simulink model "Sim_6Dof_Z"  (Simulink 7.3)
settings: Solver=ode4  StartTime=0.0  StopTime=80  FixedStep=0.0005  MaxStep=0.0005  RelTol=1e-3
InitFcn:
  | run
StopFcn:
  | Pl
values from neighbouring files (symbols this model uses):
  calfa = cos(alfa0*d2r)    [run.m]
  d2r = pi/180    (= 0.0174532925199)    [run.m]
  salfa = sin(alfa0*d2r)    [run.m]
  Thet0 = 40    [run.m]
  V0 = 18640    [run.m]
undefined symbols (not defined in the file or in its folder): Acz, Avz, Bcz, Bvz, Ccz, Cvz, Dcz, DiscIntNeverNeededParam, Dvz
libraries: simulink x4

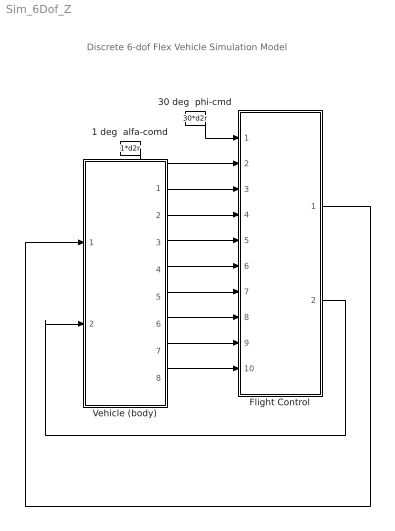
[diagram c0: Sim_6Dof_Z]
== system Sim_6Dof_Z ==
  note: Discrete 6-dof Flex Vehicle Simulation Model
  1 deg  alfa-comd : Constant  Value=1*d2r  OutDataType=sfix(16)  OutScaling=2^0
  30 deg  phi-cmd : Constant  Value=30*d2r  OutDataType=sfix(16)  OutScaling=2^0
  Flight Control : Subsystem
  Vehicle (body) : Subsystem
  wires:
  Vehicle (body)/1(phi) -> Flight Control/3(phi)
  Vehicle (body)/2(p) -> Flight Control/4(pb)
  Vehicle (body)/3(r) -> Flight Control/5(rb)
  Vehicle (body)/4(bet) -> Flight Control/6(beta)
  Vehicle (body)/5(theta) -> Flight Control/7(thet)
  Vehicle (body)/6(q) -> Flight Control/8(q)
  Vehicle (body)/7(alfa) -> Flight Control/9(alfa)
  Vehicle (body)/8(Nz) -> Flight Control/10(Nz)
  30 deg  phi-cmd/1 -> Flight Control/1(phi-cmd)
  1 deg  alfa-comd/1 -> Flight Control/2(alfa-cmd)
  Flight Control/2(Aer_pqr) -> Vehicle (body)/2(Aer_pqr)
  Flight Control/1(Jet_pqr) -> Vehicle (body)/1(Jet_pqr_Nz)

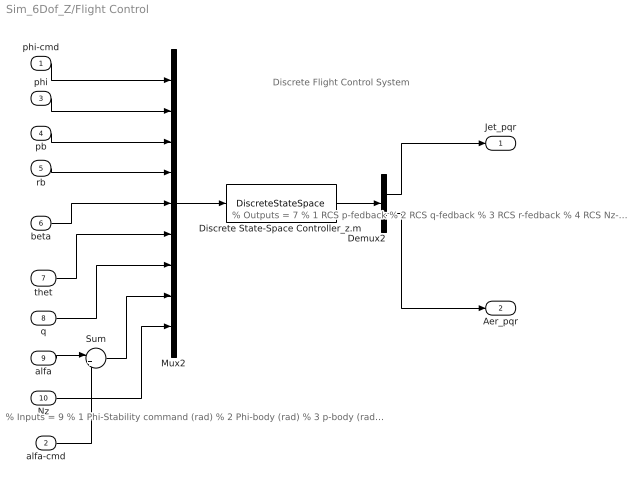
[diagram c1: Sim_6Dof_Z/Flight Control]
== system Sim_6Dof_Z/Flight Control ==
  note: Discrete Flight Control System
  note: % Outputs = 7 % 1 RCS p-fedback % 2 RCS q-fedback % 3 RCS r-fedback % 4 RCS Nz-fedback % 5 Aero-Surface p-feedback % 6 Aero-Surface q-feedback % 7 Aero-Surface r-feedback
  note: % Inputs = 9 % 1 Phi-Stability command (rad) % 2 Phi-body (rad) % 3 p-body (rad/sec) % 4 r-body (rad/sec) % 5 beta (rad) % 6 Theta (rad) % 7 q-body (rad/sec) % 8 alpha (rad) % 9 Nz (ft/sec^2)
  phi-cmd : Inport  OutDataType=sfix(16)  OutScaling=2^0
  alfa-cmd : Inport  Port=2  OutDataType=sfix(16)  OutScaling=2^0
  phi : Inport  Port=3  OutDataType=sfix(16)  OutScaling=2^0
  pb : Inport  Port=4  OutDataType=sfix(16)  OutScaling=2^0
  rb : Inport  Port=5  OutDataType=sfix(16)  OutScaling=2^0
  beta : Inport  Port=6  OutDataType=sfix(16)  OutScaling=2^0
  thet : Inport  Port=7  OutDataType=sfix(16)  OutScaling=2^0
  q : Inport  Port=8  OutDataType=sfix(16)  OutScaling=2^0
  alfa : Inport  Port=9  OutDataType=sfix(16)  OutScaling=2^0
  Nz : Inport  Port=10  OutDataType=sfix(16)  OutScaling=2^0
  Demux2 : Demux  Outputs=[4,3]
  Discrete State-Space Controller_z.m : DiscreteStateSpace  A=Acz  B=Bcz  C=Ccz  D=Dcz  SampleTime=0.04
  Mux2 : Mux  Inputs=9
  Sum : Sum  Inputs=|+-  OutDataType=sfix(16)  OutScaling=2^0
  Jet_pqr : Outport  OutDataType=sfix(16)  OutScaling=2^0
  Aer_pqr : Outport  Port=2  OutDataType=sfix(16)  OutScaling=2^0
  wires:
  Discrete State-Space Controller_z.m/1 -> Demux2/1
  Demux2/1 -> Jet_pqr/1
  Demux2/2 -> Aer_pqr/1
  phi/1 -> Mux2/2
  pb/1 -> Mux2/3
  rb/1 -> Mux2/4
  beta/1 -> Mux2/5
  thet/1 -> Mux2/6
  q/1 -> Mux2/7
  Nz/1 -> Mux2/9
  Mux2/1 -> Discrete State-Space Controller_z.m/1
  phi-cmd/1 -> Mux2/1
  alfa/1 -> Sum/1
  alfa-cmd/1 -> Sum/2
  Sum/1 -> Mux2/8

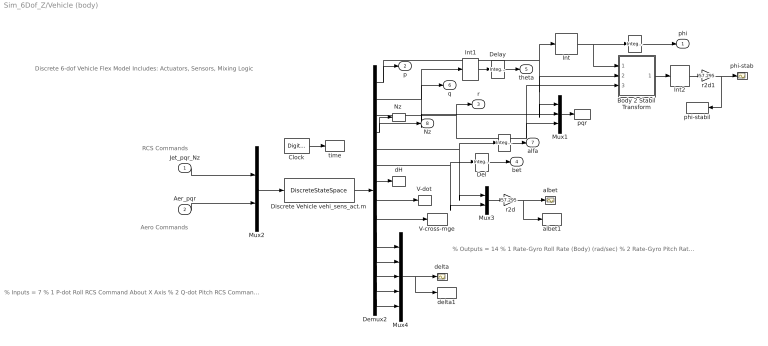
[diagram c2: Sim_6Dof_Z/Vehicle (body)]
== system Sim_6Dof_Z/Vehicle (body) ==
  note: Discrete 6-dof Vehicle Flex Model Includes: Actuators, Sensors, Mixing Logic
  note: % Outputs = 14 % 1 Rate-Gyro Roll Rate (Body) (rad/sec) % 2 Rate-Gyro Pitch Rate (Body) (rad/sec) % 3 Rate-Gyro Yaw Rate (Body) (rad/sec) % 4 Accelerom along Z, (ft/sec^2) Translat. Acceler. % 5 Angle of attack, alfa, (radians) % 6 Angle of sideslip, beta, (radian) % 7 Change in Altitude, delta-h, (feet) % 8 Forward Acceleration (V-dot) (ft/sec) % 9 Cross Range Velocity (Vcr) (ft/sec) % 10 Left Outboard Deflection (rad) % 11 Left Inboard Deflection (rad) % 12 Right Inboard Deflection (rad) % 13 Right Outboard Deflection (rad) % 14 Rudder Deflection (rad)
  note: % Inputs = 7 % 1 P-dot Roll RCS Command About X Axis % 2 Q-dot Pitch RCS Command About Y Axis % 3 R-dot Yaw RCS Command About Z Axis % 4 Az Normal Acceleration Along Z Axis % 5 P-dot Roll Aero Command About X Axis % 6 Q-dot Pitch Aero Command About Y Axis % 7 R-dot Yaw Aero Command About Z Axis
  note: RCS Commands
  note: Aero Commands
  Jet_pqr_Nz : Inport  OutDataType=sfix(16)  OutScaling=2^0
  Aer_pqr : Inport  Port=2  OutDataType=sfix(16)  OutScaling=2^0
  " " : simulink/Discrete/Integer Delay  vinit=0.0  samptime=0.04  NumDelays=1
  "  " : simulink/Discrete/Integer Delay  vinit=0.0  samptime=0.04  NumDelays=1
  Body 2 Stabil Transform : Subsystem
  Clock : DigitalClock  SampleTime=0.04
  Del : simulink/Discrete/Integer Delay  vinit=0.0  samptime=0.04  NumDelays=1
  Delay : simulink/Discrete/Integer Delay  vinit=0.0  samptime=0.04  NumDelays=1
  Demux2 : Demux  Outputs=14
  Discrete Vehicle vehi_sens_act.m : DiscreteStateSpace  A=Avz  B=Bvz  C=Cvz  D=Dvz  SampleTime=0.04
  Int : DiscreteIntegrator  SampleTime=0.04  OutDataType=sfix(16)  OutScaling=2^0  ICPrevOutput=DiscIntNeverNeededParam  ICPrevScaledInput=DiscIntNeverNeededParam
  Int1 : DiscreteIntegrator  SampleTime=0.04  OutDataType=sfix(16)  OutScaling=2^0  ICPrevOutput=DiscIntNeverNeededParam  ICPrevScaledInput=DiscIntNeverNeededParam
  Int2 : DiscreteIntegrator  SampleTime=0.04  OutDataType=sfix(16)  OutScaling=2^0  ICPrevOutput=DiscIntNeverNeededParam  ICPrevScaledInput=DiscIntNeverNeededParam
  Mux1 : Mux  Inputs=3
  Mux2 : Mux  Inputs=[4, 3]
  Mux3 : Mux  Inputs=2
  Mux4 : Mux  Inputs=5
  "Nz " : ToWorkspace  VariableName=Nz  SampleTime=-1  SaveFormat=Array
  V-cross-rnge : ToWorkspace  VariableName=Vxrng  SampleTime=-1  SaveFormat=Array
  V-dot : ToWorkspace  VariableName=dV  SampleTime=-1  SaveFormat=Array
  albet : Scope
  albet1 : ToWorkspace  VariableName=albet  SampleTime=-1  SaveFormat=Array
  dH : ToWorkspace  VariableName=dH  SampleTime=-1  SaveFormat=Array
  delta : Scope
  delta1 : ToWorkspace  VariableName=delta  SampleTime=-1  SaveFormat=Array
  phi-stab : Scope
  phi-stabil : ToWorkspace  VariableName=phi_st  SampleTime=-1  SaveFormat=Array
  pqr : ToWorkspace  VariableName=pqr  SampleTime=-1  SaveFormat=Array
  r2d : Gain  Gain=57.295  ParameterDataType=sfix(16)  ParameterScaling=2^0  OutDataType=sfix(16)  OutScaling=2^0
  r2d1 : Gain  Gain=57.295  ParameterDataType=sfix(16)  ParameterScaling=2^0  OutDataType=sfix(16)  OutScaling=2^0
  time : ToWorkspace  VariableName=time  SampleTime=-1  SaveFormat=Array
  phi : Outport  OutDataType=sfix(16)  OutScaling=2^0
  p : Outport  Port=2  OutDataType=sfix(16)  OutScaling=2^0
  r : Outport  Port=3  OutDataType=sfix(16)  OutScaling=2^0
  bet : Outport  Port=4  OutDataType=sfix(16)  OutScaling=2^0
  theta : Outport  Port=5  OutDataType=sfix(16)  OutScaling=2^0
  q : Outport  Port=6  OutDataType=sfix(16)  OutScaling=2^0
  alfa : Outport  Port=7  OutDataType=sfix(16)  OutScaling=2^0
  Nz : Outport  Port=8  OutDataType=sfix(16)  OutScaling=2^0
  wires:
  Mux2/1 -> Discrete Vehicle vehi_sens_act.m/1
  Demux2/4 -> Nz/1, "Nz "/1
  Aer_pqr/1 -> Mux2/2
  Jet_pqr_Nz/1 -> Mux2/1
  Demux2/1 -> p/1, Int/1, Mux1/1, Body 2 Stabil Transform/2(p_b)
  Demux2/2 -> q/1, Mux1/2, Int1/1
  Demux2/3 -> r/1, Mux1/3, Body 2 Stabil Transform/3(r_b)
  Demux2/14 -> Mux4/5
  Demux2/13 -> Mux4/4
  Demux2/12 -> Mux4/3
  Demux2/11 -> Mux4/2
  Demux2/10 -> Mux4/1
  Demux2/5 -> Mux3/1, " "/1
  Demux2/6 -> Mux3/2, Del/1
  Demux2/7 -> dH/1
  Demux2/8 -> V-dot/1
  Demux2/9 -> V-cross-rnge/1
  Discrete Vehicle vehi_sens_act.m/1 -> Demux2/1
  Int/1 -> Body 2 Stabil Transform/1(phi), "  "/1
  Int1/1 -> Delay/1
  Mux4/1 -> delta/1, delta1/1
  Mux1/1 -> pqr/1
  Mux3/1 -> r2d/1
  r2d/1 -> albet/1, albet1/1
  Body 2 Stabil Transform/1(p_s) -> Int2/1
  Int2/1 -> r2d1/1
  r2d1/1 -> phi-stab/1, phi-stabil/1
  Clock/1 -> time/1
  Del/1 -> bet/1
  " "/1 -> alfa/1
  "  "/1 -> phi/1
  Delay/1 -> theta/1

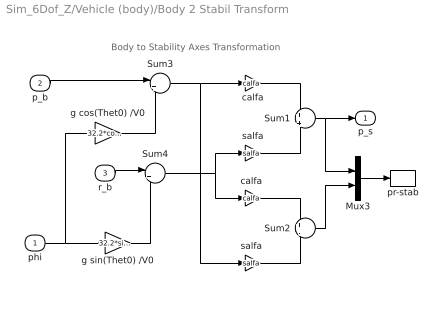
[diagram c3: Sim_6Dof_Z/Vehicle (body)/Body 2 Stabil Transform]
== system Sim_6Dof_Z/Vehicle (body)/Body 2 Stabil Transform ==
  note: Body to Stability Axes Transformation
  phi : Inport  OutDataType=sfix(16)  OutScaling=2^0
  p_b : Inport  Port=2  OutDataType=sfix(16)  OutScaling=2^0
  r_b : Inport  Port=3  OutDataType=sfix(16)  OutScaling=2^0
  Mux3 : Mux  Inputs=2
  Sum1 : Sum  Inputs=+|+  OutDataType=sfix(16)  OutScaling=2^0
  Sum2 : Sum  Inputs=+|-  OutDataType=sfix(16)  OutScaling=2^0
  Sum3 : Sum  Inputs=|++  OutDataType=sfix(16)  OutScaling=2^0
  Sum4 : Sum  Inputs=|+-  OutDataType=sfix(16)  OutScaling=2^0
  calfa : Gain  Gain=calfa  ParameterDataType=sfix(16)  ParameterScaling=2^0  OutDataType=sfix(16)  OutScaling=2^0
  "calfa " : Gain  Gain=calfa  ParameterDataType=sfix(16)  ParameterScaling=2^0  OutDataType=sfix(16)  OutScaling=2^0
  g cos(Thet0) /V0 : Gain  Gain=32.2*cos(Thet0*d2r)/V0  ParameterDataType=sfix(16)  ParameterScaling=2^0  OutDataType=sfix(16)  OutScaling=2^0
  g sin(Thet0) /V0 : Gain  Gain=32.2*sin(Thet0*d2r)/V0  ParameterDataType=sfix(16)  ParameterScaling=2^0  OutDataType=sfix(16)  OutScaling=2^0
  pr-stab : ToWorkspace  VariableName=pr_st  SampleTime=-1  SaveFormat=Array
  salfa : Gain  Gain=salfa  ParameterDataType=sfix(16)  ParameterScaling=2^0  OutDataType=sfix(16)  OutScaling=2^0
  "salfa " : Gain  Gain=salfa  ParameterDataType=sfix(16)  ParameterScaling=2^0  OutDataType=sfix(16)  OutScaling=2^0
  p_s : Outport  OutDataType=sfix(16)  OutScaling=2^0
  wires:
  "salfa "/1 -> Sum2/2
  "calfa "/1 -> Sum2/1
  salfa/1 -> Sum1/2
  calfa/1 -> Sum1/1
  Sum3/1 -> calfa/1, "salfa "/1
  Sum4/1 -> salfa/1, "calfa "/1
  phi/1 -> g sin(Thet0) /V0/1, g cos(Thet0) /V0/1
  g sin(Thet0) /V0/1 -> Sum4/2
  g cos(Thet0) /V0/1 -> Sum3/2
  r_b/1 -> Sum4/1
  p_b/1 -> Sum3/1
  Sum2/1 -> Mux3/2
  Sum1/1 -> p_s/1, Mux3/1
  Mux3/1 -> pr-stab/1
